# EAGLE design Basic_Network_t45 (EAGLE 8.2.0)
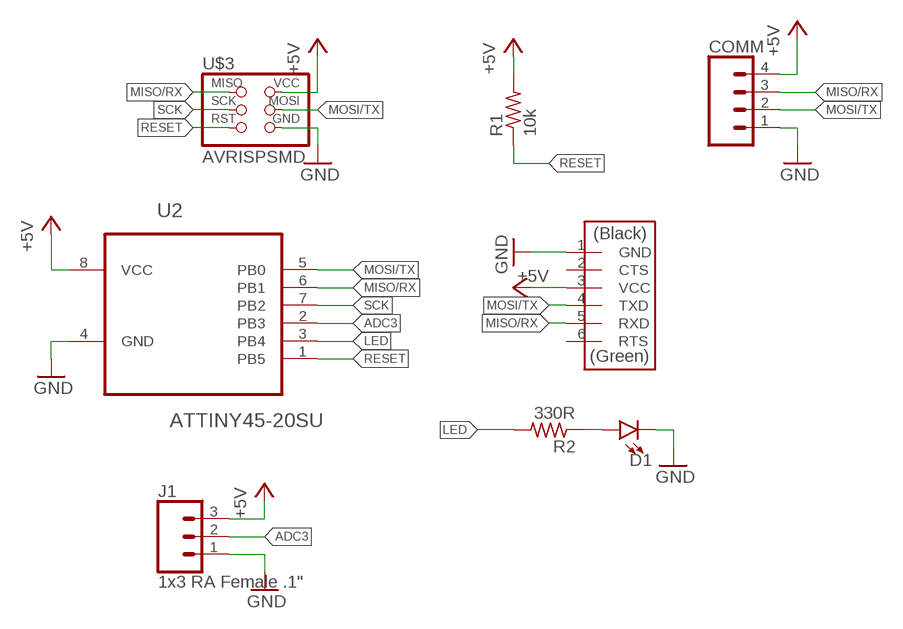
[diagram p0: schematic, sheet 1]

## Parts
COMM  CONN_04SMD_RA_FEMALE  [1X04_SMD_RA_FEMALE]
D1  LED1206  [LED-1206]
FTDI  FTDI-SMD-HEADER  [1X06SMD]
J1  1x3 RA Female .1"  CONN_03SMD_RA_MALE  [1X03_SMD_RA_MALE]
R1  10k  R-US_R1206  [R1206]
R2  330R  R-US_R1206  [R1206]
U2  ATTINY45-20SU  [SOIC127P798X216-8N]
U$3  AVRISPSMD  [2X03SMD]

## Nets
+5V: COMM.4 FTDI.3(VCC) J1.3 R1.2 U2.8(VCC) U$3.2(VCC)
ADC3: J1.2 U2.2(PB3)
GND: COMM.1 D1.C FTDI.1(GND) J1.1 U2.4(GND) U$3.6(GND)
LED: R2.2 U2.3(PB4)
MISO/RX: COMM.3 FTDI.5(RXD) U2.6(PB1) U$3.1(MISO)
MOSI/TX: COMM.2 FTDI.4(TXD) U2.5(PB0) U$3.4(MOSI)
N$4: D1.A R2.1
RESET: R1.1 U2.1(PB5) U$3.5(RST)
SCK: U2.7(PB2) U$3.3(SCK)
Unconnected: FTDI.2(CTS) FTDI.6(RTS)

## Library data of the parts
COMM = SparkFun-Connectors:CONN_04: Multi connection point. Often used as Generic Header-pin footprint for 0.1 inch spaced/style header connections On any of the 0.1 inch spaced packages, you can populate with these: Break Away Headers - Straight (PRT-00116) Break Away Male Headers - Right Angle (PRT-00553) Female Headers (PRT-00115)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
D1 = SparkFun-LED:LED: LED (Generic)
FTDI = fab:FTDI-SMD-HEADER
J1 = SparkFun-Connectors:CONN_03: Multi connection point. Often used as Generic Header-pin footprint for 0.1 inch spaced/style header connections On any of the 0.1 inch spaced packages, you can populate with these: Break Away Headers - Straight (PRT-00116) Break Away Male Headers - Right Angle (PRT-00553) Female Headers (PRT-00115)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; PROD_ID: CONN-10925
R1 R2 = rcl:R-US_: RESISTOR, American symbol
U2 = Atmel_By_element14_Batch_1-00:ATTINY45-20SU: 8-bit Microcontroller with 4 Bytes In-System Programmable Flash; MPN: ATTINY45-20SU; OC_FARNELL: 1288353; OC_NEWARK: 23M5073; PACKAGE: SOIC-8; SUPPLIER: Atmel
U$3 = fab:AVRISP

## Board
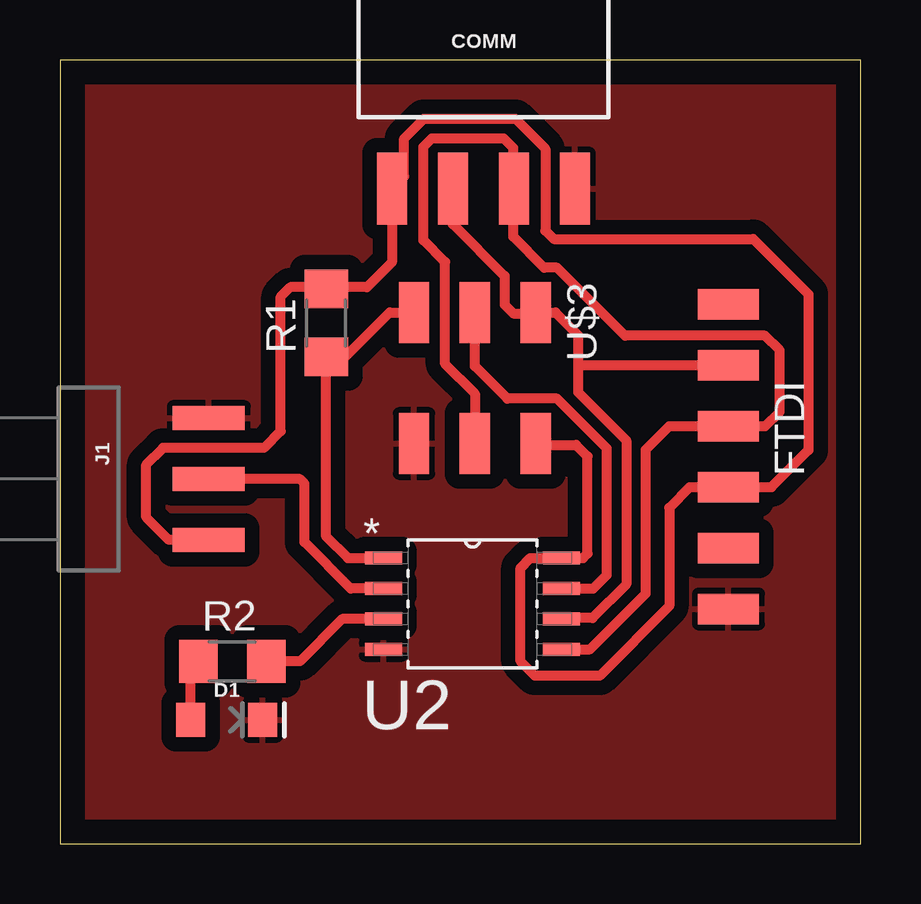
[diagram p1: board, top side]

Size 33.39 x 32.67 mm. Coordinates in mm from the lower left corner, seen from the top.
Outline: 0,0 33.39,0 33.39,32.67 0,32.67 0,0
Copper layers (1*16): Top 0.035mm / dielectric 1.5mm / Bottom 0.035mm
Design rules "default *": minimum track width 6mil, minimum drill 0.35mm, track to track 0.4mm, track to pad 0.4mm, pad to pad 0.4mm, via to via 0.4mm, smd to smd 6mil, copper to edge 40mil, drill to drill 6mil, minimum pad ring 10mil, minimum via ring 8mil, stop-mask expansion 4mil, vias tented up to drill 0mil, thermal gap 10mil

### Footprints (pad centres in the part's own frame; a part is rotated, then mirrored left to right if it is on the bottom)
1X04_SMD_RA_FEMALE = smd 1.25 x 3: 1 -3.81,7.225; 2 -1.27,7.225; 3 1.27,7.225; 4 3.81,7.225
LED-1206 = smd 1.2 x 1.4: A -1.5,0; C 1.5,0
1X06SMD = smd 2.54 x 1.27: 1 0,6.35; 2 0,3.81; 3 0,1.27; 4 0,-1.27; 5 0,-3.81; 6 0,-6.35
1X03_SMD_RA_MALE = smd 1 x 3: 1 -2.54,5; 2 0,5; 3 2.54,5
R1206 = smd 1.6 x 1.803: 1 -1.422,0; 2 1.422,0
SOIC127P798X216-8N = smd 1.549 x 0.533: 1 -3.708,1.905; 2 -3.708,0.635; 3 -3.708,-0.635; 4 -3.708,-1.905; 5 3.708,-1.905; 6 3.708,-0.635; 7 3.708,0.635; 8 3.708,1.905
2X03SMD = smd 2.54 x 1.27: 1 -2.54,2.54; 2 2.92,2.54; 3 -2.54,0; 4 2.92,0; 5 -2.54,-2.54; 6 2.92,-2.54

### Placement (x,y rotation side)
COMM  17.65,34.53 180 top
D1  6.95,5.16 0 top
FTDI  27.87,16.13 180 top
J1  1.2,15.2 270 top
R1  11.1,21.71 90 top
R2  7.19,7.6 0 top
U2  17.2,10 0 top
U$3  17.3,19.6 270 top

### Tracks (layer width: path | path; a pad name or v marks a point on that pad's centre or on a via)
+5V
  Top 0.406: U$3.2 19.9,16.62 21.52,16.62 21.99,16.14 21.99,12.09 21.8,11.9 U2.8 19.6,11.9 19.2,11.5 19.2,7.6 19.8,7 22.5,7 25.4,9.9 25.4,14 26.26,14.86 FTDI.3 29.66,14.86 31.2,16.4 31.2,22.9 28.9,25.2 20.59,25.2 20.23,25.55 20.23,28.97 18.99,30.21 15.17,30.21 14.35,29.39 14.35,27.81 COMM.4 | J1.3 4.54,12.66 3.6,13.6 3.6,15.8 4.3,16.5 8.5,16.5 9.2,17.2 9.2,22.8 9.6,23.2 11.03,23.2 | 11.03,23.2 R1.2 | 13.9,26.96 COMM.4 | COMM.4 13.84,24.24 12.8,23.2 11.03,23.2
ADC3
  Top 0.406: U2.2 12.12,10.63 10.19,12.57 10.19,15.01 10,15.2 J1.2
GND
  pour Top (isolate 0.61): 0,32.6 33.2,32.6 33.2,0 0,0
LED
  Top 0.406: U2.3 11.77,9.37 10,7.6 R2.2
MISO/RX
  Top 0.406: 19.98,22 U$3.1 | 21.6,20 21.6,18.82 23.61,16.81 23.61,10.81 22.2,9.4 20.94,9.4 U2.6 | COMM.3 16.38,25.82 18.54,23.66 18.54,22.46 18.9,22.1 19.8,22.1 U$3.1 | FTDI.5 21.66,19.94 21.6,20 | U$3.1 20.66,22.14 21.6,21.2 21.6,20
MOSI/TX
  Top 0.406: U2.5 22.1,8.1 24.41,10.41 24.41,16.41 25.4,17.4 FTDI.4 29.4,17.4 30,18 30,20.57 29.39,21.18 23.56,21.18 20.73,24.01 20.19,24.01 18.9,25.3 18.9,27.32 | U$3.4 17.3,18.76 16.06,20 16.06,24.25 15.15,25.16 15.15,29.05 15.51,29.41 18.49,29.41 18.9,29 18.9,27.32 | COMM.2 19,26.98 | 18.9,26.89 COMM.2 | 18.9,27.32 COMM.2
N$4
  Top 0.406: D1.A 5.45,7.28 R2.1
RESET
  Top 0.406: U2.1 12,11.9 11.1,12.8 R1.1 11.89,20.29 13.74,22.14 U$3.5
SCK
  Top 0.406: U$3.3 17.3,19.9 18.65,18.55 20.73,18.55 22.8,16.48 22.8,11.2 22.23,10.63 U2.7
